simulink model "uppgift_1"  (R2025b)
settings: Solver=VariableStepAuto  StartTime=0.0  StopTime=10.0  RelTol=1e-3

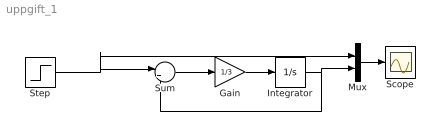
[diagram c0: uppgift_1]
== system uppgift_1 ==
  Gain : Gain  Gain=1/3
  Integrator : Integrator
  Mux : Mux  Inputs=2
  Scope : Scope
  Step : Step  SampleTime=0
  Sum : Sum  Inputs=|+-
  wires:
  Sum/1 -> Gain/1
  Gain/1 -> Integrator/1
  Mux/1 -> Scope/1
  Integrator/1 -> Sum/2, Mux/2
  Step/1 -> Sum/1, Mux/1
